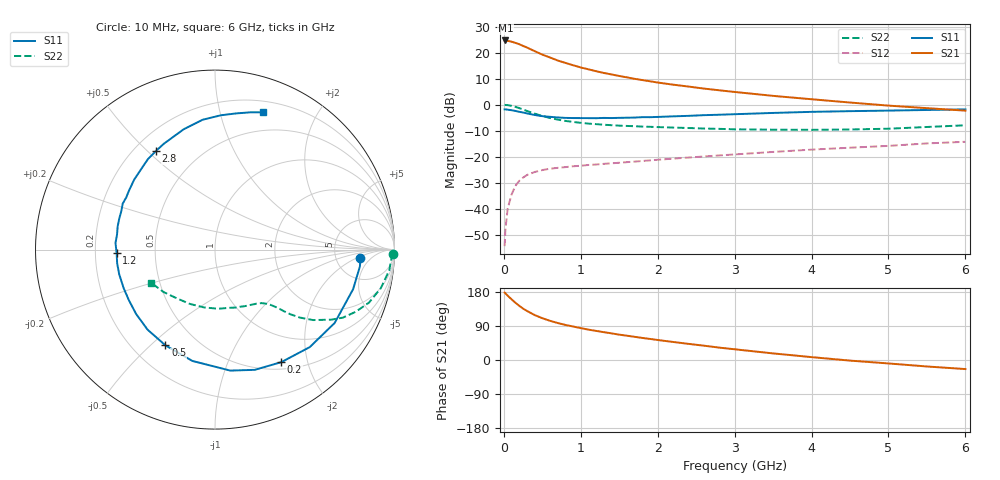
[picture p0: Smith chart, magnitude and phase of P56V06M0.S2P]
! SIEMENS Small Signal Semiconductors
! BFP183
! Si NPN RF Bipolar Junction Transistor in SOT143
! VCE = 6 V  IC = 6 mA
! Common Emitter S-Parameters:  March  1996
# GHz  S  MA  R  50
!  f  S11  S21  S12  S22
! GHz  MAG  ANG  MAG  ANG  MAG  ANG  MAG  ANG
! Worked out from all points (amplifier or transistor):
!   36 points, 10 MHz to 6 GHz, reference 50 ohm
!   highest |S21| = 24.7 dB at 20 MHz (marker M1)
!   |S21| within 3 dB of that: start of sweep to 321 MHz
!   unconditionally stable (mu >= 1): 1.513 GHz to 5.715 GHz
!   at 250 MHz: K = 0.22, MSG = 25.3 dB, |S12| = -28.0 dB
!   at 1.4 GHz: K = 0.96, MSG = 17.1 dB, |S12| = -22.6 dB
!   at 6 GHz: K = 0.96, MSG = 6.0 dB, |S12| = -14.3 dB
!   lowest NFmin = 1.20 dB at 450 MHz
!   S11 on the Smith chart (normalised r, x): 10 MHz: 8.97, -2.38; 200 MHz: 0.59, -1.59; 500 MHz: 0.33, -0.56; 1.2 GHz: 0.29, -0.02; 2.8 GHz: 0.29, +0.53; 6 GHz: 0.31, +1.37
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0.01  0.8114 -3.2  17.11 178.0  0.0019 83.1  0.9914 -1.3
0.02  0.8129 -6.6  17.15 176.2  0.0039 86.0  0.9847 -2.7
0.05  0.8005 -16.0  16.85 169.8  0.0101 82.3  0.978 -6.7
0.1  0.782 -31.5  16.24 160.2  0.0186 73.9  0.9486 -13.1
0.15  0.7576 -45.8  15.4 151.2  0.0275 66.9  0.9073 -19.0
0.2  0.7278 -59.5  14.53 143.0  0.0342 61.1  0.8576 -23.8
0.25  0.7056 -71.7  13.47 135.6  0.0396 56.4  0.8073 -28.0
0.3  0.6795 -82.8  12.56 129.6  0.0443 51.3  0.7556 -31.1
0.4  0.633 -101.5  10.69 118.6  0.0507 45.5  0.6729 -35.7
0.5  0.6007 -117.4  9.17 110.3  0.0552 40.9  0.6056 -38.7
0.6  0.5832 -130.1  8.071 103.4  0.0586 38.2  0.5537 -40.6
0.7  0.5672 -140.8  7.06 97.6  0.0609 36.3  0.5153 -41.8
0.9  0.5523 -157.2  5.727 88.4  0.0653 34.4  0.4654 -43.4
1.1  0.5505 -172.0  4.78 80.1  0.0692 33.3  0.4321 -45.1
1.2  0.5484 -178.1  4.393 76.8  0.0706 33.1  0.4218 -46.0
1.7  0.5645 157.6  3.136 61.2  0.0803 34.0  0.3847 -51.6
2.2  0.5955 139.2  2.422 47.6  0.0916 34.3  0.3623 -59.1
2.8  0.6399 121.1  1.888 32.7  0.1056 33.5  0.3424 -70.6
3.5  0.6927 104.6  1.475 17.4  0.1233 31.6  0.33 -86.6
4.5  0.7494 87.4  1.098 -1.6  0.1486 26.6  0.3332 -114.6
5.5  0.7897 75.6  0.856 -17.1  0.1797 21.5  0.3718 -140.6
6  0.8108 70.6  0.767 -23.9  0.1932 17.5  0.401 -152.6
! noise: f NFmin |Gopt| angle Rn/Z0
0.45  1.2  0.21  41  0.24
0.9  1.25  0.24  101  0.21
1.8  2  0.32  175  0.14
